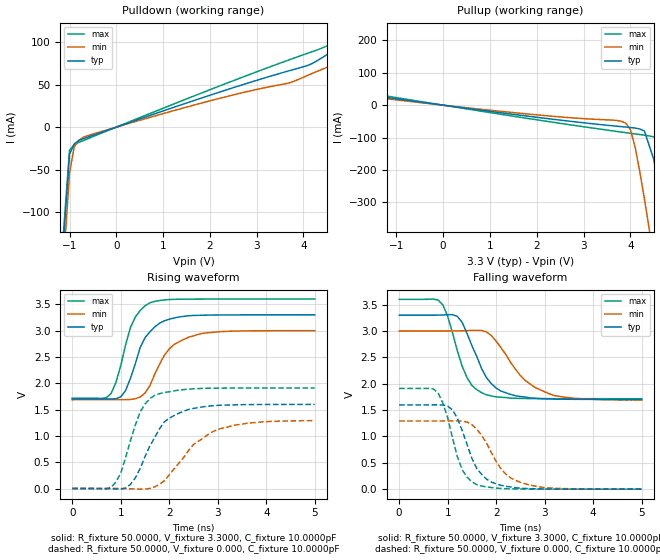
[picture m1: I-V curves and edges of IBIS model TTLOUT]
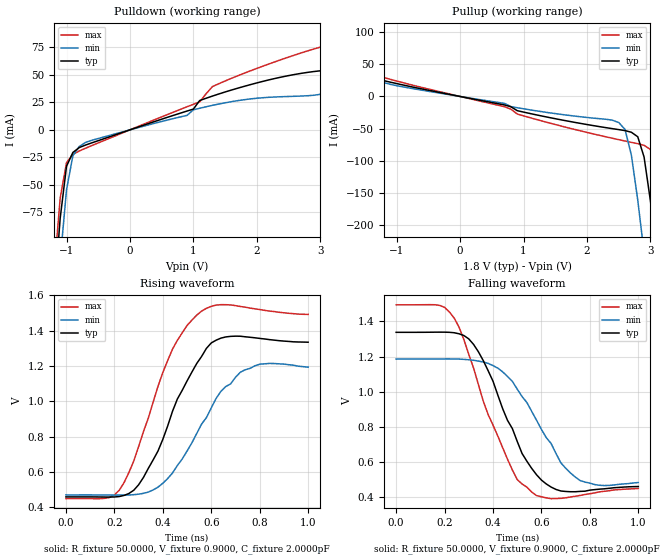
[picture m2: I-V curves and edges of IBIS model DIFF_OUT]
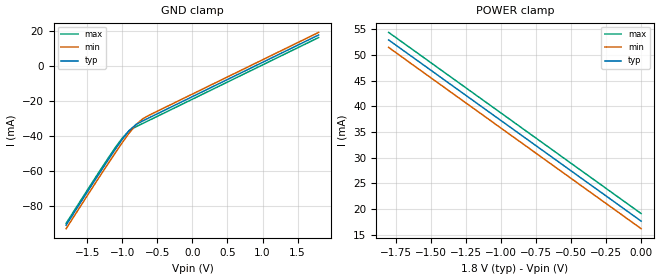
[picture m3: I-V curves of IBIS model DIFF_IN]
[IBIS ver]   2.1
[File name]   warp217_33_50.ibs
[File Rev]   1.0
[Date]   January 10, 2000
[Source]   Motorola, data from spice models.
[Notes]   This model represents the MC92600 WarpLink Quad Gigabit
   transceiver in 3.3V TTL I/O power configuration with
   50 ohm media in a 217 PBGA
[Disclaimer]   This is a preliminary model for review purposes only.
[Copyright]   Copyright 2000 Motorola Inc.
|   Component MC92600
[Component]   MC92600
[Manufacturer]   Motorola Inc.
[Package]
| variable   typ   min   max
R_pkg   0.1500   NA   NA
L_pkg   6.8000nH   NA   NA
C_pkg   1.7000pF   NA   NA
[Pin]  signal_name   model_name   R_pin   L_pin   C_pin
B3   recv_d_5   TTLOUT
C2   recv_d_4   TTLOUT
B1   recv_d_3   TTLOUT
C1   recv_d_2   TTLOUT
C3   recv_d_1   TTLOUT
D2   recv_d_0   TTLOUT
D1   recv_c_0   TTLOUT
D3   recv_c_1   TTLOUT
E2   recv_c_2   TTLOUT
E3   recv_c_3   TTLOUT
F2   recv_c_4   TTLOUT
F1   recv_c_5   TTLOUT
G2   recv_c_6   TTLOUT
F3   recv_c_7   TTLOUT
G1   recv_c_k   TTLOUT
H2   recv_c_9   TTLOUT
H1   recv_c_rclk   TTLOUT
J1   recv_c_idle   TTLOUT
H3   recv_c_err   TTLOUT
J2   recv_b_err   TTLOUT
K1   recv_b_idle   TTLOUT
K2   recv_b_rclk   TTLOUT
J3   recv_b_9   TTLOUT
L1   recv_b_k   TTLOUT
L2   recv_b_7   TTLOUT
M1   recv_b_6   TTLOUT
L3   recv_b_5   TTLOUT
M2   recv_b_4   TTLOUT
N1   recv_b_3   TTLOUT
M3   recv_b_2   TTLOUT
P1   recv_b_1   TTLOUT
P2   recv_b_0   TTLOUT
N3   recv_a_0   TTLOUT
R1   recv_a_1   TTLOUT
T1   recv_a_2   TTLOUT
P3   recv_a_3   TTLOUT
N4   recv_a_4   TTLOUT
R3   recv_a_5   TTLOUT
T2   recv_a_6   TTLOUT
T3   recv_a_7   TTLOUT
U3   recv_a_k   TTLOUT
T4   recv_a_9   TTLOUT
U4   recv_a_rclk   TTLOUT
R4   recv_a_idle   TTLOUT
R5   recv_a_err   TTLOUT
T5   xmit_b_idle_b   TTLIN
U5   xmit_b_k   TTLIN
T6   xmit_b_7   TTLIN
R6   xmit_b_6   TTLIN
U6   xmit_b_5   TTLIN
T7   xmit_b_4   TTLIN
U7   xmit_b_3   TTLIN
R7   xmit_b_2   TTLIN
T8   xmit_b_1   TTLIN
R8   xmit_b_0   TTLIN
U8   xmit_a_0   TTLIN
U10   xmit_a_1   TTLIN
T10   xmit_a_2   TTLIN
R10   xmit_a_3   TTLIN
U11   xmit_a_4   TTLIN
T11   xmit_a_5   TTLIN
R11   xmit_a_6   TTLIN
T12   xmit_a_7   TTLIN
T13   xmit_a_k   TTLIN
U13   tst_1   TTLIN
R12   wse_gen   TTLIN
T14   xmit_a_idle_b   TTLIN
U14   tst_0   TTLIN
U15   bsync_1   TTLIN
R13   bsync_0   TTLIN
R14   lbe   TTLIN
P13   lboe   TTLIN
T15   tbie   TTLIN
R16   media   TTLIN
P17   rlk_a_n   DIFF_IN
N17   rlk_a_p   DIFF_IN
N15   xlk_a_n   DIFF_OUT
M15   xlk_a_p   DIFF_OUT
M14   xlk_b_p   DIFF_OUT
L14   xlk_b_n   DIFF_OUT
L17   rlk_b_p   DIFF_IN
K17   rlk_b_n   DIFF_IN
K15   pll_tpa   NC
H17   rlk_c_n   DIFF_IN
G17   rlk_c_p   DIFF_IN
H14   xlk_c_n   DIFF_OUT
G14   xlk_c_p   DIFF_OUT
G15   xlk_d_p   DIFF_OUT
F15   xlk_d_n   DIFF_OUT
E17   rlk_d_p   DIFF_IN
D17   rlk_d_n   DIFF_IN
C16   repe   TTLIN
E14   rcce   TTLIN
C15   adie   TTLIN
B16   wse   TTLIN
B15   hse   TTLIN
C14   ddre   TTLIN
A15   ref_clk   TTLIN
B14   reset_b   TTLIN
A14   stndby   TTLIN
D13   xmit_d_idle_b   TTLIN
B13   xmit_d_k   TTLIN
A13   xmit_d_7   TTLIN
C13   xmit_d_6   TTLIN
B12   xmit_d_5   TTLIN
A12   xmit_d_4   TTLIN
B11   xmit_d_3   TTLIN
A11   xmit_d_2   TTLIN
C11   xmit_d_1   TTLIN
C10   xmit_d_0   TTLIN
B10   xmit_c_0   TTLIN
A10   xmit_c_1   TTLIN
C8   xmit_c_2   TTLIN
B8   xmit_c_3   TTLIN
A8   xmit_c_4   TTLIN
A7   xmit_c_5   TTLIN
B7   xmit_c_6   TTLIN
C7   xmit_c_7   TTLIN
A6   xmit_c_k   TTLIN
B6   xmit_c_idle_b   TTLIN
C6   recv_d_err   TTLOUT
B5   recv_d_idle   TTLOUT
A4   recv_d_rclk   TTLOUT
C5   recv_d_9   TTLOUT
C4   recv_d_k   TTLOUT
B4   recv_d_7   TTLOUT
A3   recv_d_6   TTLOUT
A1   GND   GND
H9   GND   GND
P4   GND   GND
A17   GND   GND
H10   GND   GND
P6   GND   GND
B2   GND   GND
J8   GND   GND
P8   GND   GND
D4   GND   GND
J9   GND   GND
P10   GND   GND
D6   GND   GND
J10   GND   GND
P12   GND   GND
D8   GND   GND
K4   GND   GND
P14   GND   GND
D10   GND   GND
K8   GND   GND
R15   GND   GND
D12   GND   GND
K9   GND   GND
T16   GND   GND
F4   GND   GND
K10   GND   GND
U1   GND   GND
H4   GND   GND
M4   GND   GND
U17   GND   GND
H8   GND   GND
F17   GND   GND
H15   GND   GND
J14   GND   GND
L15   GND   GND
M17   GND   GND
J16   GND   GND
C17   GND   GND
D15   GND   GND
E15   GND   GND
F14   GND   GND
J17   GND   GND
N14   GND   GND
P15   GND   GND
R17   GND   GND
T17   GND   GND
K16   GND   GND
F16   VDD18   POWER
G16   VDD18   POWER
J15   VDD18   POWER
M16   VDD18   POWER
N16   VDD18   POWER
B17   VDD18   POWER
D14   VDD18   POWER
D16   VDD18   POWER
E16   VDD18   POWER
H16   VDD18   POWER
K14   VDD18   POWER
L16   VDD18   POWER
P16   VDD33   POWER
A5   VDD33   POWER
C12   VDD33   POWER
E1   VDD33   POWER
E4   VDD33   POWER
G3   VDD33   POWER
K3   VDD33   POWER
N2   VDD33   POWER
P5   VDD33   POWER
R2   VDD33   POWER
U12   VDD33   POWER
A2   VDD18   POWER
A9   VDD18   POWER
A16   VDD18   POWER
B9   VDD18   POWER
C9   VDD18   POWER
D5   VDD18   POWER
D7   VDD18   POWER
D9   VDD18   POWER
D11   VDD18   POWER
G4   VDD18   POWER
J4   VDD18   POWER
L4   VDD18   POWER
P7   VDD18   POWER
P9   VDD18   POWER
P11   VDD18   POWER
R9   VDD18   POWER
T9   VDD18   POWER
U2   VDD18   POWER
U9   VDD18   POWER
U16   VDD18   POWER
[Diff Pin]  inv_pin  vdiff   tdelay_typ  tdelay_min  tdelay_max
N17   P17   0.2000V  NA   NA   NA
M15   N15   NA   NA   NA   NA
L17   K17   0.2000V  NA   NA   NA
M14   L14   NA   NA   NA   NA
G17   H17   0.2000V  NA   NA   NA
G14   H14   NA   NA   NA   NA
E17   D17   0.2000V  NA   NA   NA
G15   F15   NA   NA   NA   NA
| Models and submodels in the file (4): TTLOUT (Output), DIFF_OUT (Output), DIFF_IN (Input), TTLIN (Input)
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|   Model TTLOUT
[Model]   TTLOUT
Model_type   Output
Vmeas =   1.5000V
Cref =  10.0000pF
Rref =  50.0000
Vref =  0.000V
C_comp   7.0000pF   NA   NA
[Temperature Range]   40.0000   0.1050k   0.000
[Pullup Reference]   3.3000V   3.0000V   3.6000V
[Pulldown Reference]   0.000V   0.000V   0.000V
[POWER Clamp Reference]   3.3000V   3.0000V   3.6000V
[GND Clamp Reference]   0.000V   0.000V   0.000V
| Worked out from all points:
|   slope of the pulldown table from 0 to 0.495 V, typ, clamps not added: 52.2 ohm
|   slope of the pullup table from 0 to 0.495 V, typ, clamps not added: 51.8 ohm
|   rising waveform, R_fixture 50.0000, V_fixture 3.3000, C_fixture 10.0000pF: 20-80 % time 436ps typ, 502ps min, 358ps max; typ from 1.7 V to 3.3 V
|   rising waveform, R_fixture 50.0000, V_fixture 0.000, C_fixture 10.0000pF: 20-80 % time 550ps typ, 810ps min, 418ps max; typ from 0 V to 1.6 V
|   falling waveform, R_fixture 50.0000, V_fixture 3.3000, C_fixture 10.0000pF: 20-80 % time 496ps typ, 712ps min, 398ps max; typ from 3.3 V to 1.7 V
|   falling waveform, R_fixture 50.0000, V_fixture 0.000, C_fixture 10.0000pF: 20-80 % time 437ps typ, 548ps min, 356ps max; typ from 1.6 V to 0 V
[Pulldown]
| voltage   I(typ)   I(min)   I(max)
-3.3V     -2.179A    -2.215A    -2.16A
-1.5V     -425mA     -467.3mA   -401mA
-1V       -31.83mA   -54.1mA    -27.12mA
-900mV    -19.76mA   -23.33mA   -20.69mA
-700mV    -13.48mA   -11.71mA   -15.65mA
3.7V      66.34mA    52.04mA    79.19mA
4.1V      72.66mA    61.06mA    87mA
4.5V      85.05mA    70.25mA    95.28mA
5.1V      104.9mA    83.83mA    119.1mA
5.5V      116.2mA    95.61mA    136.1mA
5.9V      127.1mA    131.7mA    152.2mA
6.6V      198.6mA    445.1mA    178.5mA
[Pullup]
| voltage   I(typ)   I(min)   I(max)
-3.3V     145.6mA    240mA      128.2mA
-2.9V     64.6mA     88.22mA    70.31mA
-2.5V     49.58mA    45.39mA    58.29mA
3.8V      -66.18mA   -49.58mA   -82.93mA
4V        -68.9mA    -74.84mA   -86.83mA
4.2V      -73.41mA   -204.2mA   -90.66mA
4.3V      -79.67mA   -289mA     -92.65mA
4.5V      -167.5mA   -469.9mA   -97.65mA
4.7V      -337.3mA   -657.6mA   -110.7mA
4.9V      -522.4mA   -848.5mA   -228.4mA
5.1V      -712.6mA   -1.041A    -406.5mA
6.6V      -2.18A     -2.511A    -1.864A
[Ramp]
| variable   typ   min   max
dV/dt_r   0.9605/0.3693n   0.7767/0.5765n   1.1478/0.2664n
dV/dt_f   0.9602/0.2710n   0.7886/0.4250n   1.1323/0.1936n
R_load = 50.0000
[Rising Waveform]
R_fixture = 50.0000
V_fixture = 3.3000
V_fixture_min = 3.0000
V_fixture_max = 3.6000
C_fixture = 10.0000pF
R_dut = 0.1500
L_dut = 6.8000nH
C_dut = 1.7000pF
| time   V(typ)   V(min)   V(max)
0s        1.702V     1.687V     1.716V
800ps     1.701V     1.687V     1.804V
1ns       1.742V     1.687V     2.336V
1.2ns     2.096V     1.692V     3.061V
1.4ns     2.678V     1.739V     3.383V
1.6ns     2.977V     1.953V     3.529V
2ns       3.217V     2.652V     3.591V
2.4ns     3.282V     2.876V     3.598V
3.1ns     3.298V     2.983V     3.6V
5ns       3.3V       2.999V     3.6V
[Rising Waveform]
R_fixture = 50.0000
V_fixture = 0.000
V_fixture_min = 0.000
V_fixture_max = 0.000
C_fixture = 10.0000pF
R_dut = 0.1500
L_dut = 6.8000nH
C_dut = 1.7000pF
| time   V(typ)   V(min)   V(max)
0s        269.4nV    6.943uV    1.538uV
800ps     -3.817mV   40.15uV    20.31mV
1ns       -10.32mV   -123.1uV   291.4mV
1.2ns     79.13mV    -4.502mV   910.3mV
1.4ns     381.3mV    -12.31mV   1.456V
1.7ns     969.6mV    32.41mV    1.771V
2.1ns     1.388V     375.2mV    1.855V
2.5ns     1.522V     837.6mV    1.895V
3ns       1.58V      1.124V     1.907V
5ns       1.598V     1.29V      1.91V
[Falling Waveform]
R_fixture = 50.0000
V_fixture = 3.3000
V_fixture_min = 3.0000
V_fixture_max = 3.6000
C_fixture = 10.0000pF
R_dut = 0.1500
L_dut = 6.8000nH
C_dut = 1.7000pF
| time   V(typ)   V(min)   V(max)
0s        3.3V       3V         3.6V
700ps     3.3V       3V         3.605V
900ps     3.304V     3V         3.499V
1.2ns     3.277V     3.002V     2.623V
1.4ns     2.953V     3.007V     2.115V
1.8ns     2.116V     2.983V     1.789V
2.1ns     1.86V      2.683V     1.744V
2.5ns     1.757V     2.154V     1.721V
3ns       1.715V     1.847V     1.717V
5ns       1.702V     1.689V     1.716V
[Falling Waveform]
R_fixture = 50.0000
V_fixture = 0.000
V_fixture_min = 0.000
V_fixture_max = 0.000
C_fixture = 10.0000pF
R_dut = 0.1500
L_dut = 6.8000nH
C_dut = 1.7000pF
| time   V(typ)   V(min)   V(max)
0s        1.599V     1.293V     1.91V
800ps     1.599V     1.293V     1.831V
1ns       1.576V     1.293V     1.354V
1.1ns     1.503V     1.293V     971.1mV
1.3ns     1.112V     1.29V      368.1mV
1.6ns     393.5mV    1.137V     84.4mV
2.1ns     74.01mV    385mV      13.76mV
2.5ns     18.73mV    129.1mV    2.699mV
3.1ns     2.583mV    23.59mV    242.8uV
5ns       6.271uV    156.7uV    1.721uV
|   Model DIFF_OUT
[Model]   DIFF_OUT
Model_type   Output
Vmeas =   1.5000V
Cref =  10.0000pF
Rref =  50.0000
Vref =   0.9000V
C_comp   7.0000pF   NA   NA
[Temperature Range]   40.0000   0.1050k   0.000
[Pullup Reference]   1.8000V   1.6500V   1.9500V
[Pulldown Reference]   0.000V   0.000V   0.000V
[POWER Clamp Reference]   1.8000V   1.6500V   1.9500V
[GND Clamp Reference]   0.000V   0.000V   0.000V
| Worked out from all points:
|   slope of the pulldown table from 0 to 0.27 V, typ, clamps not added: 51.2 ohm
|   slope of the pullup table from 0 to 0.27 V, typ, clamps not added: 52.2 ohm
|   rising waveform, R_fixture 50.0000, V_fixture 0.9000, C_fixture 2.0000pF: 20-80 % time 172ps typ, 186ps min, 158ps max; typ from 0.458 V to 1.33 V
|   falling waveform, R_fixture 50.0000, V_fixture 0.9000, C_fixture 2.0000pF: 20-80 % time 161ps typ, 183ps min, 165ps max; typ from 1.34 V to 0.462 V
[Pulldown]
| voltage   I(typ)   I(min)   I(max)
-1.8V     -710.4mA   -751.2mA   -687.8mA
-1.2V     -156.1mA   -198.2mA   -132.8mA
-1.1V     -80.36mA   -118.3mA   -61.99mA
-1V       -33.11mA   -54.48mA   -29.75mA
-900mV    -20.55mA   -23.58mA   -22.39mA
-800mV    -16.11mA   -15.16mA   -19.21mA
1.1V      26.61mA    19.58mA    25.42mA
1.3V      30.63mA    22.22mA    39.24mA
3.1V      54.1mA     34.7mA     76.65mA
3.3V      55.15mA    54.04mA    79.64mA
3.4V      55.97mA    84.13mA    81.04mA
3.6V      65.11mA    199.2mA    83.68mA
[Pullup]
| voltage   I(typ)   I(min)   I(max)
-1.8V     56.14mA    106mA      52.98mA
-1.6V     38.62mA    43.74mA    42.31mA
-1.4V     30.25mA    28.94mA    35.02mA
2.4V      -50.19mA   -36.98mA   -65.16mA
2.6V      -53.19mA   -51.45mA   -69.47mA
2.7V      -55.84mA   -91.88mA   -71.57mA
2.8V      -62.83mA   -161.6mA   -73.64mA
2.9V      -94.55mA   -243.9mA   -76.18mA
3.1V      -246.3mA   -422.7mA   -113.2mA
3.2V      -335.5mA   -515.5mA   -183.3mA
3.3V      -427.5mA   -609.5mA   -268.2mA
3.6V      -711.8mA   -896mA     -546.1mA
[Ramp]
| variable   typ   min   max
dV/dt_r   0.5955/0.1077n   0.4861/0.1967n   0.6857/63.9208p
dV/dt_f   0.5247/75.2612p   0.4722/0.1643n   0.6291/47.5695p
R_load = 50.0000
[Rising Waveform]
R_fixture = 50.0000
V_fixture = 0.9000
V_fixture_min = 0.8250
V_fixture_max = 0.9750
C_fixture = 2.0000pF
R_dut = 0.1500
L_dut = 6.8000nH
C_dut = 1.7000pF
| time   V(typ)   V(min)   V(max)
0s        457.9mV    469.1mV    448.3mV
220ps     459.9mV    468.1mV    495.3mV
300ps     526.5mV    473.4mV    743.1mV
400ps     784.1mV    535.3mV    1.163V
460ps     1.013V     635.7mV    1.345V
560ps     1.254V     870.4mV    1.511V
620ps     1.346V     1.016V     1.545V
720ps     1.369V     1.165V     1.537V
820ps     1.353V     1.212V     1.516V
1ns       1.335V     1.193V     1.492V
[Falling Waveform]
R_fixture = 50.0000
V_fixture = 0.9000
V_fixture_min = 0.8250
V_fixture_max = 0.9750
C_fixture = 2.0000pF
R_dut = 0.1500
L_dut = 6.8000nH
C_dut = 1.7000pF
| time   V(typ)   V(min)   V(max)
0s        1.338V     1.186V     1.494V
180ps     1.339V     1.187V     1.491V
240ps     1.336V     1.187V     1.419V
340ps     1.227V     1.175V     1.04V
380ps     1.12V      1.161V     870.8mV
480ps     791.1mV    1.059V     556mV
560ps     564.7mV    888.6mV    430.7mV
680ps     436.7mV    597.1mV    394.8mV
760ps     434.5mV    495.8mV    411.4mV
1ns       462.2mV    484.8mV    451mV
|   Model DIFF_IN
[Model]   DIFF_IN
Model_type   Input
Vinl = 0.7000V
Vinh = 1.1000V
C_comp   7.0000pF   NA   NA
[Temperature Range]   40.0000   0.1050k   0.000
[Pullup Reference]   1.8000V   1.6500V   1.9500V
[Pulldown Reference]   0.000V   0.000V   0.000V
[POWER Clamp Reference]   1.8000V   1.6500V   1.9500V
[GND Clamp Reference]   0.000V   0.000V   0.000V
[GND_clamp]
| voltage   I(typ)   I(min)   I(max)
-1.8V     -91.18mA   -93.2mA    -90.14mA
-1.3V     -59.92mA   -62mA      -58.86mA
-1V       -42.1mA    -43.99mA   -41.33mA
-900mV    -36.96mA   -38.41mA   -37.1mA
-800mV    -33.48mA   -33.5mA    -34.81mA
-700mV    -31.38mA   -30.11mA   -32.84mA
1.8V      17.65mA    19.12mA    16.18mA
[POWER_clamp]
| voltage   I(typ)   I(min)   I(max)
-1.8V     52.94mA    51.49mA    54.41mA
-1.7V     50.98mA    49.52mA    52.45mA
-1.5V     47.06mA    45.59mA    48.53mA
0V        17.65mA    16.18mA    19.12mA
